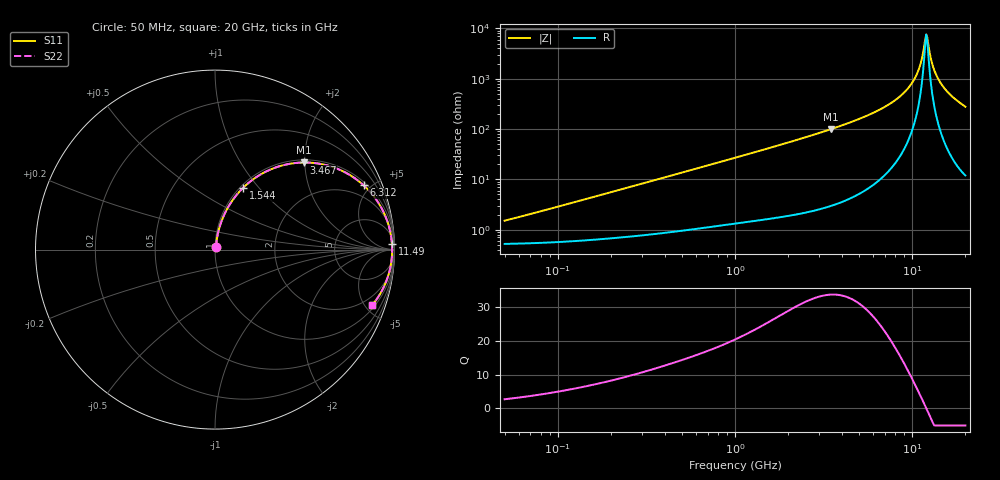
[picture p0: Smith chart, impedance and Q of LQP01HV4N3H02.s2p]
!Murata Part Number: LQP01HV4N3H02
!These Parameters are Measured in Series Mode Connection
!  o--[Z]--o
!Port1  Port2
!  o-------o
!Freq. Start=50[MHz] Stop=20[GHz], 401[Steps]
# Hz S RI R 50
!Freq.(Hz) S11(Real) S11(Imag) S21(Real) S21(Imag) S12(Real) S12(Imag) S22(Real) S22(Imag)
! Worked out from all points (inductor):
!   401 points, 50 MHz to 20 GHz, reference 50 ohm
!   read as one part in series: L = 4.49 nH near 56.37 MHz
!   highest Q = 33.6 at 3.467 GHz (marker M1), where L = 4.54 nH
!   self-resonance near 12.02 GHz
!   S11 on the Smith chart (normalised r, x): 50 MHz: 1.01, +0.03; 1.544 GHz: 1.03, +0.83; 3.467 GHz: 1.06, +1.98; 6.312 GHz: 1.17, +4.53; 11.49 GHz: 25, +55; 20 GHz: 1.24, -5.55
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5e7  0.00537 0.014  0.9946 -0.014  0.9946 -0.014  0.00537 0.014
1.364002e8  0.00744 0.0376  0.9926 -0.0376  0.9926 -0.0376  0.00744 0.0376
3.721004e8  0.0182 0.0987  0.9818 -0.0987  0.9818 -0.0987  0.0182 0.0987
1e9  0.0774 0.2437  0.9226 -0.2437  0.9226 -0.2437  0.0774 0.2437
1.544007e9  0.156 0.3438  0.844 -0.3438  0.844 -0.3438  0.156 0.3438
2.728004e9  0.3662 0.4665  0.6338 -0.4665  0.6338 -0.4665  0.3662 0.4665
3.466789e9  0.4945 0.4853  0.5055 -0.4853  0.5055 -0.4853  0.4945 0.4853
4.677679e9  0.669 0.4552  0.331 -0.4552  0.331 -0.4552  0.669 0.4552
6.311513e9  0.8276 0.3589  0.1724 -0.3589  0.1724 -0.3589  0.8276 0.3589
7.442007e9  0.8962 0.2819  0.1038 -0.2819  0.1038 -0.2819  0.8962 0.2819
8.774992e9  0.9468 0.1923  0.0532 -0.1923  0.0532 -0.1923  0.9468 0.1923
9.892087e9  0.9712 0.1217  0.0288 -0.1217  0.0288 -0.1217  0.9712 0.1217
1.082228e10  0.9823 0.0668  0.0177 -0.0668  0.0177 -0.0668  0.9823 0.0668
1.115139e10  0.9845 0.0482  0.0155 -0.0482  0.0155 -0.0482  0.9845 0.0482
1.149051e10  0.9861 0.0295  0.0139 -0.0295  0.0139 -0.0295  0.9861 0.0295
1.183995e10  0.9869 0.0107  0.0131 -0.0107  0.0131 -0.0107  0.9869 0.0107
1.201863e10  0.987 0.00133  0.013 -0.00133  0.013 -0.00133  0.987 0.00133
1.220001e10  0.987 -0.00808  0.013 0.00808  0.013 0.00808  0.987 -0.00808
1.314879e10  0.9841 -0.0552  0.0159 0.0552  0.0159 0.0552  0.9841 -0.0552
1.438523e10  0.9744 -0.1117  0.0256 0.1117  0.0256 0.1117  0.9744 -0.1117
1.646126e10  0.9467 -0.1951  0.0533 0.1951  0.0533 0.1951  0.9467 -0.1951
2e10  0.875 -0.3099  0.125 0.3099  0.125 0.3099  0.875 -0.3099
